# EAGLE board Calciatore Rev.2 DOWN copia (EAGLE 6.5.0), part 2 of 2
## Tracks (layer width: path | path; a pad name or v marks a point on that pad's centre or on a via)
3.3V  (via drill 0.6, 0.9 pad 1.68)  (4 unrouted)
  Top 0.305: 25.76,91.66 C23.1 | 207.73,96.14 R2.2 | C24.1 152.65,135.63 | 94.83,136.49 v94.7,136.36
  Top 0.813: C6.1 184.33,93.38 DX.BW | 207.73,96.14 207.73,97.37 v209,98.64 | v182.97,127.22 183.6,126.58 v183.6,116.42 182.53,115.35 182.53,107.91 C58.+ | v182.97,139.28 182.97,142.46 | 182.97,142.46 v182.97,144.36 | 182.97,142.46 181.7,142.46 v175.35,148.81 | v175.35,148.81 174.58,149.57 151.22,149.57 v150.84,149.95 125.69,149.95 v125.18,149.44 | 152.65,135.63 154.39,137.38 163.92,137.38 v175.35,148.81 | v125.82,142.46 124.55,141.19 v118.2,141.19 | v113.75,136.11 v106.39,136.11 106.13,135.85 106.13,133.92 | 106.13,133.92 104.5,133.92 | 104.5,133.92 102.32,136.11 99.15,136.11 | 94.83,136.49 98.77,136.49 99.15,136.11 | 104.5,133.92 104.7,133.72 C25.1 106.13,133.92 | 99.15,136.11 v99.15,130.39 | v104.23,129.12 v108.04,129.12 | v83.65,139.41 v83.65,142.2 | v80.1,142.46 74.98,142.46 AX.BW | v42.63,146.9 v40.09,149.44 38.82,149.44 v31.84,142.46 | v29.3,127.85 28.03,126.58 v28.03,124.68 | SX.BW 25.26,116.2 22.95,113.88 v22.95,106.9 22.95,106.04 25.49,103.5 | SX.VCC 25.49,103.5 | 25.49,103.5 25.26,103.5 23.58,101.82 23.58,94.66 | 23.58,94.66 C23.1 | 23.58,94.66 17.06,94.66 12.79,90.39 12.79,89.04 D11.2 | D12.2 12.86,71.9 18.5,66.26 18.5,60.54 25.49,53.56 39.46,53.56 | 39.46,53.56 44.94,53.56 v45.36,53.97 | v45.36,51.43 v45.36,53.97 | v45.36,53.97 v45.36,56.51 v45.36,59.05 | v65.49,34.51 42.63,34.51 37.55,39.59 37.55,51.65 39.46,53.56 | 154.71,67.21 148.04,73.88 142.96,73.88 139.15,77.69 139.15,86.58 138.09,87.64 PDX.VDD 112.91,87.64 TEENSY3.2_1.3.3V1 | PWR.3 158.51,71.01 154.71,67.21 | 154.71,67.21 152.87,65.37 v152.87,58.89 | PX.BW 98.7,24.53 99.78,25.62 99.78,44.67 v97.88,46.57 | v97.24,54.19 TEENSY3.2_1.3.3V
  Top 0.813: v64.22,85.94 64.22,77.64 63.87,77.28 63.87,75.6 IC2.24
  Top 1: U$10.VOUT 184.22,92.34 C6.1
  Bottom 0.305: R39.2 166.06,64.59 PWR.3 | ASX.VDD 75.1,127.13 | 196.44,107.8 R37.2 195.03,107.8 | 152.84,58.61 v152.87,58.89 | 28.03,143.73 28.03,144.04 R19.2 | 184.24,146.27 184.95,146.27 R33.2 | 83.27,144.33 R49.2 | 106.18,137.42 R23.2 106.13,138.01 | 117.56,143.38 R25.2
  Bottom 0.813: U$10.VOUT 184.22,68.78 183.6,68.16 183.6,65.38 R39.2 | DX.BW 187,98.42 182.66,102.76 182.66,102.78 182.53,102.91 182.53,107.87 C58.+ | 195.03,107.8 191.71,111.12 DX.VCC 191,111.12 193.13,113.25 193.13,116.42 | v209,98.64 209.64,99.28 209.64,110.71 203.92,116.42 193.13,116.42 | v183.6,116.42 193.13,116.42 | R35.2 183.8,128.05 | 183.8,128.05 v182.97,127.22 | 183.8,128.05 183.8,138.45 v182.97,139.28 | v182.97,144.36 183.05,144.36 R33.2 | v175.35,148.81 174.08,150.08 174.08,162.17 R31.2 | v150.84,149.95 150.84,152.29 R29.2 | v125.18,149.44 125.18,143.09 v125.82,142.46 129.63,142.46 130.26,143.09 130.26,144.97 R27.2 | R25.2 117.56,143.61 117.56,141.82 v118.2,141.19 118.2,140.55 v113.75,136.11 | v106.39,136.11 106.39,137.22 106.18,137.42 | R51.2 94.7,142.3 v94.7,136.36 86.7,136.36 v83.65,139.41 | v99.15,130.39 100.42,129.12 v104.23,129.12 | v108.04,129.12 109.31,130.39 119.47,130.39 | 119.47,130.39 124.55,130.39 135.34,119.6 136.39,119.6 ADX.VDD | QUANTUM_CONNECTOR.26 120.21,129.65 119.47,130.39 | v83.65,142.2 83.65,143.73 | 83.65,143.73 83.65,143.95 83.27,144.33 | v80.1,142.46 82,142.46 83.27,143.73 83.65,143.73 | AX.BW 74.57,142.91 72.48,145 63.99,145 AX.VCC 57.83,146.9 v42.63,146.9 | 64.23,145.23 R47.2 | R21.2 38.7,159.72 40.09,158.33 v40.09,149.44 | v31.84,142.46 29.61,142.46 | 29.61,142.46 R19.2 | 29.61,142.46 29.61,128.16 v29.3,127.85 | R17.2 22.17,124.68 v28.03,124.68 28.03,117.92 SX.BW | v22.95,106.9 20.99,106.9 R15.2 | D11.2 D13.2 D30.2 D6.2 D12.2 | v45.36,59.05 45.36,59.72 42,63.08 32.85,63.08 R13.2 | R45.2 64.45,30.92 66.13,32.6 66.13,33.87 v65.49,34.51 | 152.84,58.61 R41.2
  Bottom 0.813: v97.88,46.57 97.24,47.21 v97.24,54.19 | PX.BW 98.7,22.26 99.15,21.81 109.31,21.81 | 109.31,21.81 109.71,21.81 PX.VCC | R43.2 108.78,21.28 109.31,21.81 | 73.75,142.05 73.75,128.98 ASX.VDD | 75.1,127.13 74.93,127.13 73.11,125.31 73.11,111.34 77.56,106.9 77.56,96.1 76.92,95.47 75.69,95.47 PSX.VDD 68.58,95.38 64.22,91.02 v64.22,85.94
5V  (via drill 0.6)
  Top 0.305: QUANTUM_CONNECTOR.25 120.21,123.3 147.41,96.1 147.41,92.13 C15.+
  Top 0.813: v180.43,72.61 181.7,72.61 187.41,78.32 v195.67,78.32 | v198.21,94.2 198.21,94.83 199.48,96.1 201.47,96.1 R3.2
  Bottom 0.813: 158.39,77.24 IC1.3 158.39,81.15 C15.+ | 158.39,77.24 156.93,75.78 155.03,75.78 153.76,74.51 153.76,72.46 PWR.1 | 158.39,77.24 170.08,77.24 174.71,72.61 v180.43,72.61 | v195.67,78.32 196.3,78.32 198.21,80.23 v198.21,94.2
BATLVL  (via drill 0.6)
  Top 0.305: TP1.TP 205.99,72.77 203.92,70.7 171.54,70.7 171.54,70.57 149.69,48.73 | 149.69,48.73 98.26,48.73 95.97,51.02 v95.97,59.91 | TEENSY3.2_1.32 104.67,74.51 102.96,74.51 101.56,73.11 96.35,73.11 94.7,71.46 94.7,65.24 v95.34,64.61 | R6.2 133.32,73.48 R5.1 136.97,72.89 138.52,71.34 146.14,71.34 149.31,68.16 149.69,67.78 149.69,48.73
  Bottom 0.305: v95.34,64.61 95.34,63.72 95.97,63.08 v95.97,59.91
BLUE(RGB)  (via drill 0.6)
  Top 0.305: v128.99,129.76 127.09,129.76 125.18,127.85 115.02,127.85 113.88,126.71 113.88,122.26 108.67,117.06 90.26,117.06 v89.62,116.42 | v143.6,141.19 147.77,141.19 R-B.1
  Bottom 0.305: v128.99,129.76 140.42,141.19 v143.6,141.19 | v89.62,116.42 89.62,115.15 106.13,98.64 107.4,98.64 120.1,85.94 120.1,67.53 119.47,66.89 115.02,66.89 TEENSY3.2_1.5
BUZZER
  Bottom 0.305: TEENSY3.2_1.RESET/DAC 102.32,84.67 102.32,91.02 87.08,106.26 86.45,106.26 80.1,99.91 80.1,94.83 79.46,94.2 79.46,82.13 76.29,78.96 75.02,78.96 74.38,79.59 74.38,87.21 72.07,89.53 BUZZER.+
CS1
  Top 0.305: IC2.22 66.31,77.24 68.67,79.59 68.67,85.94 72.48,89.75 72.48,118.33 73.75,119.6 75.51,119.6 ASX.CS
CS2  (via drill 0.6)
  Top 0.305: IC2.21 67.58,76.6 69.3,78.32 69.3,85.31 73.11,89.12 73.11,106.26 v73.75,106.9 | v71.21,106.9 71.84,107.53 71.84,118.96 74.38,121.5 74.38,127.85 74.94,128.41 78.12,128.41 80.73,131.03 80.73,135.47 82.64,137.38 107.4,137.38 108.04,138.01 135.34,138.01 139.79,133.57 139.79,130.14 ADX.CS
  Bottom 0.305: v73.75,106.9 v71.21,106.9
CS3  (via drill 0.6)
  Top 0.305: IC2.20 68.85,76.6 69.94,77.69 69.94,84.67 73.75,88.48 73.75,90.39 75.02,91.66 76.29,91.66 78.83,94.2 78.83,99.91 85.18,106.26 85.18,108.8 v91.53,115.15 | PDX.CS 135.8,96.1 v134.07,96.1
  Bottom 0.305: v134.07,96.1 133.44,96.74 110.58,96.74 108.04,99.28 106.77,99.28 91.53,114.52 v91.53,115.15
CS4
  Top 0.305: IC2.19 70.12,76.6 70.57,77.05 70.57,84.04 74.38,87.85 75.52,87.85 PSX.CS
D+
  Bottom 0.305: USB_2.3 84.54,32.6 87.72,35.78 104.23,35.78 106.13,37.68 USB.2
D-
  Bottom 0.305: USB.1 103.59,37.68 102.32,36.41 87.08,36.41 82,31.33 USB_2.2
EXP-READ-1  (via drill 0.6)
  Top 0.305: TEENSY3.2_1.14/A0 99.59,82.13 v83.91,82.13 | v80.1,75.15 v80.1,68.16 | v69.3,68.16 68.03,69.43 66.76,69.43 64.86,67.53 64.22,67.53 63.77,67.08 IC2.1
  Bottom 0.305: v83.91,82.13 82.64,80.86 82.64,78.96 80.1,76.42 v80.1,75.15 | v80.1,68.16 79.46,67.53 69.3,67.53 v69.3,68.16
EXPA
  Top 0.305: IC2.10 75.2,63.72 75.96,62.95 96.1,62.95 98.51,60.54 100.42,60.54 101.05,59.91 101.05,58.64 102.96,56.73 111.21,56.73 111.85,57.37 111.85,58.64 112.48,59.27 114.83,59.27 TEENSY3.2_1.2
EXPB
  Top 0.305: IC2.11 76.47,64.35 77.23,63.59 97.37,63.59 98,62.95 113.69,62.95 TEENSY3.2_1.3
EXPC  (via drill 0.6)
  Top 0.305: IC2.14 76.47,74.33 v77.56,73.24 | v102.96,75.78 108.67,75.78 109.05,75.78 109.31,75.78 111.21,73.88 111.21,70.07 112.48,68.8 112.48,66.26 114.48,64.25 TEENSY3.2_1.4
  Bottom 0.305: v77.56,73.24 100.42,73.24 v102.96,75.78
EXPD  (via drill 0.6)
  Top 0.305: TEENSY3.2_1.24 107.4,71.97 108.67,71.97 109.94,70.7 109.94,64.99 109.31,64.35 105.5,64.35 102.96,66.89 v102.32,66.89 | IC2.13 78.65,76.42 80.73,76.42 82,75.15 v82,68.16 | v101.69,69.43 101.69,70.07 101.05,70.7 v95.97,70.7
  Bottom 0.305: v102.32,66.89 101.69,67.53 v101.69,69.43 | v82,68.16 82.64,67.53 93.43,67.53 95.97,70.07 v95.97,70.7
GND  (via drill 0.6, 1.1)
  Top 0.305: v112.48,40.22 112.48,39.59 111.21,38.32 USB.3 | C25.2 108.73,132.99 108.17,132.99 106.89,131.71 102.91,131.71 101.05,133.57 v101.05,134.76
  Top 0.406: v72.48,80.86 75.19,78.14 IC2.15
  Bottom 0.305: C51.2 63.22,28.49 62.72,28.99 62.72,31.53 C52.1 | TEENSY3.2_1.GND 108.57,51.55 108.04,50.38 108.04,44.67 v112.48,40.22 | v101.05,134.76 101.05,136.74 99.78,138.01 98.51,138.01 97.24,139.28 97.24,142.51 C22.1 | C29.1 117.87,146.06 C28.2
  Bottom 0.406: BUZZER.- 59.33,88.3 65.49,82.13 71.21,82.13 v72.48,80.86
  other vias: 45.43,48.98 45.43,46.57 45.43,43.9 45.43,41.24
  pour Top (isolate 0.406): -25.31,195.8 245.83,192.62 245.83,-21.37 -25.31,-18.2
  pour Bottom (isolate 0.406): -19.6,197.07 258.53,195.8 258.53,-19.47 -19.6,-18.2
GREEN(RGB)  (via drill 0.6)
  Top 0.305: v127.09,132.93 114.64,132.93 108.8,127.09 108.8,122.26 104.86,118.33 v85.18,118.33 | v138.52,146.9 147.91,146.9 R-G.1
  Bottom 0.305: v127.09,132.93 137.25,143.09 137.25,145.63 v138.52,146.9 | v85.18,118.33 85.18,117.06 104.86,97.37 106.13,97.37 118.83,84.67 118.83,71.97 116.19,69.33 TEENSY3.2_1.6
INA1-31-2
  Top 0.305: ASX.INA 75.59,111.92 77.56,113.88 77.56,123.41 82,127.85 87.93,127.85 QUANTUM_CONNECTOR.2
INA2-32-2
  Top 0.305: ADX.INA 112.88,134.6 109.31,131.03 102.32,131.03 QUANTUM_CONNECTOR.8
INA3-33-2
  Bottom 0.305: 136.43,103.09 PDX.INA 135.77,102.88 135.34,102.45 135.34,99.28 134.71,98.64 112.48,98.64 109.94,101.18 108.67,101.18 94.7,115.15 94.7,115.79 QUANTUM_CONNECTOR.11
INA4-34-2  (via drill 0.6)
  Top 0.305: QUANTUM_CONNECTOR.5 | QUANTUM_CONNECTOR.5 90.89,119.6 80.73,119.6 80.1,118.96 80.1,113.25 83.91,109.44 v83.91,108.8
  Bottom 0.305: 84.54,108.8 v83.91,108.8 85.18,107.53 85.18,106.26 79.46,100.55 79.46,95.47 78.83,94.83 78.83,83.4 75.61,80.18 PSX.INA
INB1-35-2
  Top 0.305: QUANTUM_CONNECTOR.6 94.81,127.74 93.43,129.12 80.12,129.12 ASX.INB
INB2-36-2
  Bottom 0.305: ADX.INB 134.31,121.9 122.64,133.57 115.66,133.57 113.75,131.66 108.67,131.66 104.86,127.85 104.23,127.85 QUANTUM_CONNECTOR.12
INB3-37-2
  Bottom 0.305: 136.43,90.39 PDX.INB 135.34,91.48 135.34,96.74 134.71,97.37 111.21,97.37 108.67,99.91 107.4,99.91 92.8,114.52 92.8,118.96 QUANTUM_CONNECTOR.7
INB4-38-2
  Top 0.305: PSX.INB 75.61,92.88 78.19,95.47 78.19,121.5 81.37,124.68 88.57,124.68 QUANTUM_CONNECTOR.1
LED1  (via drill 0.6)
  Top 0.305: LED4.A 119.62,3.87 118.83,4.66 v118.83,7.84 | 115.02,77.05 TEENSY3.2_1.9 116.1,75.78 v121.37,75.78 | v125.18,58 125.18,75.15 v124.55,75.78
  Bottom 0.305: v118.83,7.84 118.83,51.65 v125.18,58 | v124.55,75.78 v121.37,75.78
LED2  (via drill 0.6)
  Top 0.305: LED2.A 124.39,3.87 122.64,2.12 120.1,2.12 117.56,4.66 v117.56,5.93 | TEENSY3.2_1.10 116.73,77.69 122.64,77.69 123.28,77.05 v123.28,58
  Bottom 0.305: v117.56,5.93 117.56,8.47 118.2,9.11 118.2,52.92 v123.28,58
LED_ALIM  (via drill 0.6)
  Top 0.305: TEENSY3.2_1.31 106.13,78.32 109.94,78.32 111.85,76.42 111.85,70.7 114.39,68.16 v122.01,68.16 | R8.1 127.25,68.96 v127.09,68.8
  Bottom 0.305: v127.09,68.8 122.64,68.8 v122.01,68.16
MISO_12  (via drill 0.6)
  Top 0.305: v27.39,73.88 43.9,73.88 48.98,78.96 60.41,78.96 v61.05,79.59 | v86.45,104.36 100.42,104.36 110.58,94.2 v110.58,91.02
  Bottom 0.305: D12.3 15.52,73.88 v27.39,73.88 | v61.05,79.59 64.86,79.59 65.49,78.96 73.75,78.96 74.38,78.32 76.92,78.32 80.1,81.5 80.1,93.56 80.73,94.2 80.73,99.28 85.81,104.36 v86.45,104.36 | v110.58,91.02 111.21,91.02 115.02,87.21 115.02,84.67 TEENSY3.2_1.12
MOSI_11  (via drill 0.6)
  Top 0.305: v40.73,70.7 42,70.7 49.62,78.32 v62.32,78.32 | v85.81,102.45 85.18,103.09 85.18,104.99 85.81,105.63 87.08,105.63 87.72,104.99 101.05,104.99 111.85,94.2 111.85,90.39 v110.58,89.12
  Bottom 0.305: D11.3 18,88.98 36.28,70.7 v40.73,70.7 | v62.32,78.32 73.11,78.32 73.75,77.69 77.56,77.69 80.73,80.86 80.73,92.93 81.37,93.56 81.37,98.01 v85.81,102.45 | v110.58,89.12 111.85,89.12 113.75,87.21 113.75,83.21 TEENSY3.2_1.11
MOTORE1-1
  Bottom 2.184: X1.1 41.34,113.13 ASX.INMOT2
MOTORE1-2
  Bottom 2.184: X1.2 41.42,118.13 ASX.INMOT1
MOTORE2-1
  Bottom 2.184: PDX.INMOT2 166.77,101.61 X2.1
MOTORE2-2
  Bottom 2.184: PDX.INMOT1 166.75,96.53 X2.2
MOTORE3-1
  Bottom 2.184: ADX.INMOT2 166.48,133.33 X3.1
MOTORE3-2
  Bottom 2.184: ADX.INMOT1 166.5,128.25 X3.2
MOTORE4-1
  Bottom 2.184: X4.1 41.41,81.51 PSX.INMOT2
MOTORE4-2
  Bottom 2.184: X4.2 41.33,86.51 PSX.INMOT1
N$1
  Top 0.305: R1.2 LED2.C
N$2  (via drill 0.6)
  Top 0.305: R8.2 139.95,68.8 146.77,68.8 v148.04,67.53 | v167.12,63.51 173.44,69.84 204.33,69.84 207.73,73.24 207.73,84.93 LED1.A
  Bottom 0.305: v148.04,67.53 151.85,63.72 166.91,63.72 v167.12,63.51
N$3
  Bottom 0.305: 0°.VCC 103.51,148.41 C26.1 R23.1
N$4
  Bottom 0.305: R24.1 110.01,142.96 0°.OUT
N$6
  Bottom 0.305: 12°.VCC 114.91,151.03 C28.1 114.82,146.52 R25.1
N$7
  Bottom 0.305: 12°.OUT 123,146.77 R26.1
N$9
  Bottom 0.305: R13.1 C1.1 28.66,57.37 26.7,57.37 240°.VCC
N$13
  Bottom 0.305: 270°.VCC 14.19,103.37 C4.1 R15.1
N$14
  Bottom 0.305: 282°.VCC 16.95,123.48 C9.1 R17.1
N$15
  Bottom 0.305: 25°.OUT 135.4,149.25 R28.1
N$16
  Bottom 0.305: R30.1 154.39,158.97 38°.OUT
N$17
  Top 1: C5.+ 180.54,87.48 179.16,88.86 179.16,90.14 U$10.VIN U$10.SHDN 176.01,89.58 D2.C
N$18
  Bottom 0.305: 51°.OUT 182.97,162.14 R32.1
N$20
  Bottom 0.305: 25°.VCC 127.17,154.39 C30.1 127.23,148.36 R27.1
N$24
  Bottom 0.305: 295°.VCC 20.81,146.09 C11.1 R19.1
N$25
  Bottom 0.305: 308°.VCC 31.3,163.54 C13.1 R21.1
N$26
  Bottom 0.305: 321°.VCC 61.53,160.31 C17.1 61.43,155.01 R47.1
N$27
  Bottom 0.305: R34.1 191.86,143.73 194.4,145 64°.OUT
N$28
  Bottom 0.305: R29.1 C32.1 148.08,162.52 38°.VCC
N$34
  Bottom 0.305: R36.1 198.84,124.04 77°.OUT
N$35
  Bottom 0.305: 51°.VCC 177.89,168.49 C34.1 R31.1
N$36
  Bottom 0.305: R40.1 185.51,57.37 120°.OUT
N$37
  Bottom 0.305: 64°.VCC 188.68,151.35 C36.1 R33.1
N$38
  Bottom 0.305: 180°.OUT 103.17,14.14 R44.1
N$39
  Bottom 0.305: 77°.VCC 196.94,131.66 C38.1 R35.1
N$40
  Bottom 0.305: R38.1 200.53,102.69 90°.OUT
N$41
  Bottom 0.305: 90°.VCC 202.25,110.44 C43.1 195.84,110.44 R37.1
N$42
  Bottom 0.305: 150°.OUT 150.58,24.35 R42.1
N$43
  Bottom 0.305: 120°.VCC 189.95,64.35 C45.1 R39.1
N$44
  Bottom 0.305: R46.1 57.24,28.79 210°.OUT
N$45
  Bottom 0.305: 150°.VCC 157.57,26.03 157.57,28.79 C47.1 R41.1
N$51
  Bottom 0.305: R14.1 24.85,64.35 240°.OUT
N$52
  Bottom 0.305: 180°.VCC 111.62,13.78 C49.1 111.58,16.47 R43.1
N$53
  Bottom 0.305: 270°.OUT 14.13,111.44 R16.1
N$54
  Bottom 0.305: 210°.VCC 64.86,24.98 C51.1 R45.1
N$56
  Bottom 0.305: 282°.OUT R18.1
N$57
  Bottom 0.305: 295°.OUT R20.1
N$60
  Bottom 0.305: 308°.OUT 38.19,168.49 R22.1
N$64
  Top 0.305: 3.3V.A 207.74,93.19 R2.1
N$65
  Bottom 0.305: 321°.OUT 69.62,159.46 R48.1
N$67
  Top 0.305: LED_RGB.3 152.1,142.2 R-B.2
N$68
  Top 0.305: LED_RGB.1 152.26,145.6 R-G.2
N$69
  Top 0.305: R7.2 LED4.C
N$81
  Top 0.305: LED_RGB.2 150.91,143.9 R-R.2
N$95
  Top 0.305: C14.+ 149.75,82.92 IC1.1 153.25,79.31 153.25,78.19
  Top 0.813: 153.25,78.19 155.66,75.78 164.85,75.78 D1.C
N$97
  Top 0.305: 5V.A 201.59,93.19 R3.1
N$135  (via drill 0.9 pad 1.68)
  other vias: 75.84,41.27
N$136  (via drill 0.9 pad 1.68)
  other vias: 75.84,43.81
N$137  (via drill 0.9 pad 1.68)
  other vias: 75.84,46.35
N$138  (via drill 0.9 pad 1.68)
  other vias: 75.84,48.89
N$139  (via drill 0.9 pad 1.68)
  other vias: 75.84,51.43
N$140  (via drill 0.9 pad 1.68)
  other vias: 75.84,53.97
N$141  (via drill 0.9 pad 1.68)
  other vias: 75.84,56.51
N$142  (via drill 0.9 pad 1.68)
  other vias: 75.84,59.05
N$143  (via drill 0.9 pad 1.68)
  other vias: 98.51,14.85
N$144  (via drill 0.9 pad 1.68)
  other vias: 98.51,17.39
N$145  (via drill 0.9 pad 1.68)
  other vias: 98.51,19.93
N$146  (via drill 0.9 pad 1.68)
  other vias: 95.97,19.93
N$147  (via drill 0.9 pad 1.68)
  other vias: 95.97,17.39
N$148  (via drill 0.9 pad 1.68)
  other vias: 95.97,14.85
N$149  (via drill 0.9 pad 1.68)
  other vias: 70.76,59.05
N$150  (via drill 0.9 pad 1.68)
  other vias: 73.3,59.05
N$151  (via drill 0.9 pad 1.68)
  other vias: 73.3,56.51
N$152  (via drill 0.9 pad 1.68)
  other vias: 70.76,56.51
N$153  (via drill 0.9 pad 1.68)
  other vias: 70.76,53.97
N$154  (via drill 0.9 pad 1.68)
  other vias: 73.3,53.97
N$155  (via drill 0.9 pad 1.68)
  other vias: 73.3,51.43
N$156  (via drill 0.9 pad 1.68)
  other vias: 70.76,51.43
N$157  (via drill 0.9 pad 1.68)
  other vias: 70.76,48.89
N$158  (via drill 0.9 pad 1.68)
  other vias: 73.3,48.89
N$159  (via drill 0.9 pad 1.68)
  other vias: 73.3,46.35
N$160  (via drill 0.9 pad 1.68)
  other vias: 70.76,46.35
N$161  (via drill 0.9 pad 1.68)
  other vias: 70.76,43.81
N$162  (via drill 0.9 pad 1.68)
  other vias: 73.3,43.81
N$163  (via drill 0.9 pad 1.68)
  other vias: 73.3,41.27
N$165  (via drill 0.9 pad 1.68)
  other vias: 70.76,41.27
N$171  (via drill 0.9 pad 1.68)
  other vias: 68.22,41.27
N$172  (via drill 0.9 pad 1.68)
  other vias: 68.22,43.81
N$173  (via drill 0.9 pad 1.68)
  other vias: 68.22,46.35
N$174  (via drill 0.9 pad 1.68)
  other vias: 68.22,48.89
N$175  (via drill 0.9 pad 1.68)
  other vias: 68.22,51.43
N$176  (via drill 0.9 pad 1.68)
  other vias: 68.22,53.97
N$177  (via drill 0.9 pad 1.68)
  other vias: 68.22,56.51
N$178  (via drill 0.9 pad 1.68)
  other vias: 68.22,59.05
N$179  (via drill 0.9 pad 1.68)
  other vias: 93.43,14.85
N$180  (via drill 0.9 pad 1.68)
  other vias: 93.43,17.39
N$181  (via drill 0.9 pad 1.68)
  other vias: 93.43,19.93
N$182  (via drill 0.9 pad 1.68)
  other vias: 90.89,19.93
N$183  (via drill 0.9 pad 1.68)
  other vias: 90.89,17.39
N$184  (via drill 0.9 pad 1.68)
  other vias: 90.89,14.85
N$185  (via drill 0.9 pad 1.68)
  other vias: 65.68,59.05
N$186  (via drill 0.9 pad 1.68)
  other vias: 65.68,56.51
N$187  (via drill 0.9 pad 1.68)
  other vias: 65.68,53.97
N$188  (via drill 0.9 pad 1.68)
  other vias: 65.68,51.43
N$189  (via drill 0.9 pad 1.68)
  other vias: 65.68,48.89
N$190
  Bottom 0.305: 334°.VCC 80.79,150.52 C19.1 80.89,147.95 R49.1
N$191
  Bottom 0.305: 347°.VCC 92.32,147.24 C21.1 92.32,142.72 R51.1
N$192  (via drill 0.9 pad 1.68)
  other vias: 65.68,46.35
N$193  (via drill 0.9 pad 1.68)
  other vias: 65.68,43.81
N$194  (via drill 0.9 pad 1.68)
  other vias: 65.68,41.27
N$197  (via drill 0.9 pad 1.68)
  other vias: 88.35,14.85
N$198  (via drill 0.9 pad 1.68)
  other vias: 88.35,17.39
N$199  (via drill 0.9 pad 1.68)
  other vias: 88.35,19.93
N$201
  Bottom 0.305: 334°.OUT 88.77,153.6 R50.1
N$202
  Bottom 0.305: R52.1 100.25,151.21 arc90 347°.OUT
N$203  (via drill 0.9 pad 1.68)
  other vias: 85.81,19.93
N$204  (via drill 0.9 pad 1.68)
  other vias: 85.81,17.39
N$205  (via drill 0.9 pad 1.68)
  other vias: 85.81,14.85
N$207  (via drill 0.9 pad 1.68)
  other vias: 60.6,59.05
N$208  (via drill 0.9 pad 1.68)
  other vias: 63.14,59.05
N$209  (via drill 0.9 pad 1.68)
  other vias: 63.14,56.51
N$210  (via drill 0.9 pad 1.68)
  other vias: 60.6,56.51
N$211  (via drill 0.9 pad 1.68)
  other vias: 60.6,53.97
N$214  (via drill 0.9 pad 1.68)
  other vias: 63.14,53.97
N$215  (via drill 0.6)
  Top 0.305: v196.3,58.64 166.23,28.57 109.66,28.57 R4.1 | v202.65,101.82 196.14,101.82 DX.TX
  Bottom 0.305: v196.3,58.64 196.3,66.89 201.38,71.97 204.56,71.97 205.19,72.61 205.19,99.28 v202.65,101.82
N$216  (via drill 0.9 pad 1.68)
  other vias: 63.14,51.43
N$217  (via drill 0.9 pad 1.68)
  other vias: 60.6,51.43
N$218  (via drill 0.9 pad 1.68)
  other vias: 60.6,48.89
N$219  (via drill 0.9 pad 1.68)
  other vias: 63.14,48.89
N$220  (via drill 0.9 pad 1.68)
  other vias: 63.14,46.35
N$221  (via drill 0.9 pad 1.68)
  other vias: 60.6,46.35
N$222  (via drill 0.9 pad 1.68)
  other vias: 60.6,43.81
N$223  (via drill 0.9 pad 1.68)
  other vias: 63.14,43.81
N$224  (via drill 0.9 pad 1.68)
  other vias: 63.14,41.27
N$226  (via drill 0.9 pad 1.68)
  other vias: 60.6,41.27
N$235  (via drill 0.9 pad 1.68)
  other vias: 58.06,41.27
N$236  (via drill 0.9 pad 1.68)
  other vias: 58.06,43.81
N$237  (via drill 0.9 pad 1.68)
  other vias: 58.06,46.35
N$238  (via drill 0.9 pad 1.68)
  other vias: 58.06,48.89
N$241  (via drill 0.9 pad 1.68)
  other vias: 58.06,51.43
N$242  (via drill 0.9 pad 1.68)
  other vias: 58.06,53.97
N$243  (via drill 0.9 pad 1.68)
  other vias: 58.06,56.51
N$244  (via drill 0.9 pad 1.68)
  other vias: 58.06,59.05
N$245  (via drill 0.9 pad 1.68)
  other vias: 83.27,14.85
N$246  (via drill 0.9 pad 1.68)
  other vias: 83.27,17.39
N$247  (via drill 0.9 pad 1.68)
  other vias: 83.27,19.93
N$248  (via drill 0.9 pad 1.68)
  other vias: 80.73,19.93
N$249  (via drill 0.9 pad 1.68)
  other vias: 80.73,17.39
N$250  (via drill 0.9 pad 1.68)
  other vias: 80.73,14.85
N$251  (via drill 0.9 pad 1.68)
  other vias: 55.52,59.05
N$252  (via drill 0.9 pad 1.68)
  other vias: 55.52,56.51
N$253  (via drill 0.9 pad 1.68)
  other vias: 55.52,53.97
N$254  (via drill 0.9 pad 1.68)
  other vias: 55.52,51.43
N$255  (via drill 0.9 pad 1.68)
  other vias: 55.52,48.89
N$256  (via drill 0.9 pad 1.68)
  other vias: 55.52,46.35
N$257  (via drill 0.9 pad 1.68)
  other vias: 55.52,43.81
N$258  (via drill 0.9 pad 1.68)
  other vias: 55.52,41.27
N$263  (via drill 0.9 pad 1.68)
  other vias: 52.98,41.27
N$264  (via drill 0.9 pad 1.68)
  other vias: 52.98,43.81
N$265  (via drill 0.9 pad 1.68)
  other vias: 52.98,46.35
N$266  (via drill 0.9 pad 1.68)
  other vias: 52.98,48.89
N$267  (via drill 0.9 pad 1.68)
  other vias: 52.98,51.43
N$268  (via drill 0.9 pad 1.68)
  other vias: 52.98,53.97
N$269  (via drill 0.9 pad 1.68)
  other vias: 52.98,56.51
N$270  (via drill 0.9 pad 1.68)
  other vias: 52.98,59.05
N$271  (via drill 0.9 pad 1.68)
  other vias: 78.19,14.85
N$272  (via drill 0.9 pad 1.68)
  other vias: 78.19,17.39
N$273  (via drill 0.9 pad 1.68)
  other vias: 78.19,19.93
N$315  (via drill 0.9 pad 1.68)
  other vias: 75.65,19.93
N$316  (via drill 0.9 pad 1.68)
  other vias: 75.65,17.39
N$317  (via drill 0.9 pad 1.68)
  other vias: 75.65,14.85
N$318  (via drill 0.9 pad 1.68)
  other vias: 50.44,59.05
N$319  (via drill 0.9 pad 1.68)
  other vias: 50.44,56.51
N$320  (via drill 0.9 pad 1.68)
  other vias: 50.44,53.97
N$321  (via drill 0.9 pad 1.68)
  other vias: 50.44,51.43
N$322  (via drill 0.9 pad 1.68)
  other vias: 50.44,48.89
N$323  (via drill 0.9 pad 1.68)
  other vias: 50.44,46.35
N$324  (via drill 0.9 pad 1.68)
  other vias: 50.44,43.81
N$325  (via drill 0.9 pad 1.68)
  other vias: 50.44,41.27
N$330  (via drill 0.9 pad 1.68)
  other vias: 47.9,41.27
N$331  (via drill 0.9 pad 1.68)
  other vias: 47.9,43.81
N$332  (via drill 0.9 pad 1.68)
  other vias: 47.9,46.35
N$333  (via drill 0.9 pad 1.68)
  other vias: 47.9,48.89
N$334  (via drill 0.9 pad 1.68)
  other vias: 47.9,51.43
N$335  (via drill 0.9 pad 1.68)
  other vias: 47.9,53.97
N$336  (via drill 0.9 pad 1.68)
  other vias: 47.9,56.51
N$337  (via drill 0.9 pad 1.68)
  other vias: 47.9,59.05
N$338  (via drill 0.9 pad 1.68)
  other vias: 73.11,14.85
N$339  (via drill 0.9 pad 1.68)
  other vias: 73.11,17.39
N$340  (via drill 0.9 pad 1.68)
  other vias: 73.11,19.93
N$341  (via drill 0.9 pad 1.68)
  other vias: 70.57,19.93
N$342  (via drill 0.9 pad 1.68)
  other vias: 70.57,17.39
N$343  (via drill 0.9 pad 1.68)
  other vias: 70.57,14.85
NC
  Top 0.305: TEENSY3.2_1.8 TEENSY3.2_1.7
PROGRAM  (via drill 0.6)
  Top 0.305: v107.4,35.78 109.94,35.78 114.39,40.22 114.39,41.49 113.75,42.13 106.59,42.13 v105.95,42.76
  Bottom 0.305: TEENSY3.2_1.PGM 104.77,84.08 105.95,82.89 v105.95,42.76 | USB_2.5 89.62,34.51 90.26,35.14 106.77,35.14 v107.4,35.78
PWM1-2
  Top 0.305: QUANTUM_CONNECTOR.4 92.27,127.74 91.53,128.49 81.37,128.49 76.92,124.04 76.92,118.3 ASX.PWM
PWM2-2
  Top 0.305: ADX.PWM 136.47,129.52 132.04,133.95 113.5,133.95 109.94,130.39 102.96,130.39 99.78,127.22 99.78,126.16 QUANTUM_CONNECTOR.10
PWM3-2
  Bottom 0.305: PDX.PWM 136.43,98.01 111.85,98.01 109.31,100.55 108.04,100.55 93.43,115.15 93.43,117.06 QUANTUM_CONNECTOR.9
PWM4-2  (via drill 0.6)
  Top 0.305: QUANTUM_CONNECTOR.3 92.27,122.24 90.26,120.23 80.1,120.23 79.46,119.6 79.46,112.61 82.64,109.44 82.64,108.17 v83.91,106.9
  Bottom 0.305: PSX.PWM 76.2,85.22 78.19,87.21 78.19,95.47 78.83,96.1 78.83,101.82 v83.91,106.9
RED(RGB)  (via drill 0.6)
  Top 0.305: R-R.1 v140.03,143.97 | v128.74,131.66 125.82,131.66 125.18,132.3 116.29,132.3 111.34,127.34 111.34,122.26 106.77,117.69 87.72,117.69 v87.08,117.06 | v111.21,68.16 110.58,68.8 110.58,73.24 109.31,74.51 107.4,74.51 TEENSY3.2_1.25
  Bottom 0.305: v128.74,131.66 128.99,131.66 138.52,141.19 138.52,142.46 v140.03,143.97 | v87.08,117.06 87.08,116.42 105.5,98.01 106.77,98.01 119.47,85.31 119.47,70.07 117.56,68.16 v111.21,68.16
S1-A0  (via drill 0.6)
  Top 0.305: TEENSY3.2_1.15/A1 101.05,80.86 101.05,82.77 100.42,83.4 98.51,83.4 98.51,85.94 102.32,89.75 107.4,89.75 108.04,90.39 v108.04,93.56
  Bottom 0.305: R24.2 C27.1 111.58,135.84 109.31,133.57 80.1,133.57 79.46,132.93 79.46,118.96 104.86,93.56 v108.04,93.56
S2-A1  (via drill 0.6)
  Top 0.305: v106.77,94.83 106.77,91.02 106.13,90.39 101.69,90.39 v95.97,84.67
  Bottom 0.305: R26.2 C29.2 122.97,143.42 112.48,132.93 80.73,132.93 80.1,132.3 80.1,119.6 104.86,94.83 v106.77,94.83 | v95.97,84.67 95.97,78.32 97.34,76.95 TEENSY3.2_1.16/A2
S3-A2  (via drill 0.6)
  Top 0.305: v105.5,96.1 105.5,91.66 104.86,91.02 100.42,91.02 v99.78,90.39
  Bottom 0.305: R28.2 C31.2 135.59,143.97 132.8,141.19 122.01,141.19 113.12,132.3 81.37,132.3 80.73,131.66 80.73,120.23 104.86,96.1 v105.5,96.1 | TEENSY3.2_1.17/A3 101.05,75.78 101.05,89.75 100.42,90.39 v99.78,90.39
S4-A3  (via drill 0.6)
  Top 0.305: TEENSY3.2_1.18/A4 102.35,71.87 103.59,73.11 v108.8,73.11 | v117.56,73.24 v122.01,73.24
  Bottom 0.305: R30.2 C33.2 155.96,128.49 137.88,110.41 137.88,76.29 134.83,73.24 v122.01,73.24 | v108.8,73.11 109.18,73.24 v117.56,73.24
S5-A4  (via drill 0.6)
  Top 0.305: v104.86,61.81 v108.67,61.81
  Bottom 0.305: R32.2 C35.2 178.02,149.44 138.52,109.94 138.52,68.16 134.71,64.35 125.18,64.35 124.55,64.99 117.56,64.99 115.66,63.08 110.58,63.08 109.31,61.81 v108.67,61.81 | TEENSY3.2_1.19/A5 99.69,68.89 100.32,68.89 101.05,68.16 101.05,66.26 101.69,65.62 102.96,65.62 103.59,64.99 103.59,63.72 104.86,62.45 v104.86,61.81
S6-A5  (via drill 0.6)
  Top 0.305: v133.94,65.49 v137.88,65.49 | TEENSY3.2_1.20/A6 100.86,65.62 102.96,65.62 104.86,63.72 110.58,63.72 111.08,64.22 v111.08,65.49
  Bottom 0.305: R34.2 C37.2 171.12,141.4 139.15,109.44 139.15,66.76 v137.88,65.49 | v133.94,65.49 v111.08,65.49
S7-A6  (via drill 0.6)
  Top 0.305: v104.35,59.27 v108.67,59.27
  Bottom 0.305: R36.2 C42.2 174.95,122.63 172.93,120.61 151.6,120.61 139.79,108.8 139.79,65.62 136.61,62.45 118.07,62.45 116.16,60.54 113.75,60.54 112.48,59.27 v108.67,59.27 | TEENSY3.2_1.21/A7 100.86,63.08 102.96,63.08 103.46,62.57 103.46,60.16 v104.35,59.27
S8-A7  (via drill 0.6)
  Top 0.305: v97.37,56.55 v97.37,58.76 | v103.46,57.87 v110.58,57.87
  Bottom 0.305: v103.46,57.87 100.92,55.33 97.98,55.33 97.37,55.94 v97.37,56.55 | v97.37,58.76 97.37,59.4 TEENSY3.2_1.22/A8 | v110.58,57.87 115.66,57.87 119.59,61.81 137.25,61.81 140.42,64.99 140.42,93.56 141.06,94.2 146.77,94.2 147.41,94.83 147.41,97.37 148.68,98.64 162.01,98.64 163.54,97.12 163.54,93.94 173.06,93.94 174.58,95.47 190.59,95.47 195.7,100.58 C44.2 198.38,104.85 R38.2
S9-A8  (via drill 0.6)
  Top 0.305: IC2.9 73.93,63.08 74.69,62.32 95.72,62.32 98.77,59.27 99.59,59.27 TEENSY3.2_1.23/A9 99.69,58.73 105.5,52.92 v108.67,52.92
  Bottom 0.305: R40.2 C46.2 123.32,59.95 116.29,52.92 v108.67,52.92
S10-A9  (via drill 0.6)
  Top 0.305: IC2.8 72.66,62.45 73.42,61.68 92.42,61.68 94.07,60.03 94.07,47.84 97.88,44.03 v97.88,33.24 | v144.87,30.06 144.23,29.43 111.85,29.43 110.58,30.7 104.23,30.7 v101.69,33.24
  Bottom 0.305: R42.2 C48.2 148.13,30.06 v144.87,30.06 | v97.88,33.24 v101.69,33.24
S11-A10  (via drill 0.6)
  Top 0.305: IC2.7 71.39,61.81 72.15,61.05 91.91,61.05 93.43,59.53 93.43,47.21 96.61,44.03 v96.61,25.62
  Bottom 0.305: R44.2 103.32,18.95 C50.2 100.43,19.28 99.78,18.63 97.88,18.63 97.24,19.27 97.24,24.98 v96.61,25.62
S12-A11  (via drill 0.6)
  Top 0.305: IC2.6 70.12,61.18 70.88,60.41 91.4,60.41 92.8,59.02 92.8,46.57 95.34,44.03 v95.34,37.68
  Bottom 0.305: R46.2 C52.2 64,37.05 94.7,37.05 v95.34,37.68
S13-A12  (via drill 0.6)
  Top 0.305: IC2.5 68.85,63.27 v68.67,63.08
  Bottom 0.305: R14.2 C2.2 32.79,69.11 35.65,66.26 43.9,66.26 45.81,64.35 67.4,64.35 v68.67,63.08
S14-A13
  Bottom 0.305: R16.2 C8.2 24.25,111.5 25.13,112.38 30.16,112.38 33.74,108.8 33.74,75.78 36.28,73.24 40.73,73.24 48.98,64.99 88.99,64.99 96.3,57.82 100.26,57.82 100.92,58.48 100.92,60.41 TEENSY3.2_1.A10
S15-A14
  Bottom 0.305: R18.2 C10.2 27.86,125.95 29.93,125.95 34.38,121.5 34.38,76.42 36.92,73.88 41.36,73.88 49.62,65.62 100.86,65.62 TEENSY3.2_1.A11
S16-A15  (via drill 0.6)
  Top 0.305: TEENSY3.2_1.A12 105.94,68.16 v97.5,68.16
  Bottom 0.305: R20.2 C12.2 30.37,147.73 35.01,143.09 35.01,77.05 37.55,74.51 42,74.51 50.25,66.26 95.59,66.26 v97.5,68.16
S17-A16
  Bottom 0.305: R22.2 C16.2 42.63,164.37 42.63,162.78 41.9,162.04 41.9,149.34 35.65,143.09 35.65,77.69 38.19,75.15 42.63,75.15 50.89,66.89 94.07,66.89 97.88,70.7 102.32,70.7 103.59,69.43 103.59,67.53 104.32,66.79 TEENSY3.2_1.A13
S18-A17
  Bottom 0.305: R48.2 69.72,152.16 C18.2 69.72,151.57 77.56,143.73 77.56,117.06 108.67,85.94 108.67,77.69 108.04,77.05 107.4,77.05 TEENSY3.2_1.26
S19-A18  (via drill 0.6)
  Top 0.305: v109.94,79.59 107.4,79.59 TEENSY3.2_1.27
  Bottom 0.305: R50.2 88.87,144.94 C20.1 88.87,143.61 86.45,141.19 79.46,141.19 78.19,139.28 78.19,117.69 109.31,86.58 110.58,86.58 111.21,85.94 111.21,80.23 110.58,79.59 v109.94,79.59 | 107.4,79.59 TEENSY3.2_1.27
S20-A19  (via drill 0.6)
  Top 0.305: v92.16,140.55 v99.78,140.55 | v109.31,92.29 109.31,90.39 108.04,89.12 106.77,89.12 105.98,88.33 105.98,83.36 TEENSY3.2_1.28
  Bottom 0.305: R52.2 97.45,145.52 C22.2 100.25,141.02 v99.78,140.55 | v92.16,140.55 80.1,140.55 78.83,138.65 78.83,118.33 104.86,92.29 v109.31,92.29
SCK_13  (via drill 0.6)
  Top 0.305: v42,69.43 50.25,77.69 60.41,77.69 v61.05,77.05
  Bottom 0.305: D13.3 20.53,85.18 36.28,69.43 v42,69.43 | v61.05,77.05 62.95,77.05 63.59,77.69 71.84,77.69 72.48,77.05 78.19,77.05 81.37,80.23 81.37,92.29 82,92.93 82,97.37 85.81,101.18 90.89,101.18 98.51,93.56 98.51,85.75 TEENSY3.2_1.13
SCL_29  (via drill 0.6)
  Top 0.305: v45.17,66.89 45.17,70.07 51.52,76.42 57.24,76.42 58.51,75.15 v58.51,74.51 | v102.32,77.24 101.05,75.78 v97.88,75.78
  Bottom 0.305: D6.3 25.61,77.56 36.28,66.89 v45.17,66.89 | v58.51,74.51 62.95,74.51 64.86,76.42 70.57,76.42 71.21,75.78 77.56,75.78 79.46,73.88 95.97,73.88 v97.88,75.78 | TEENSY3.2_1.29 104.67,82.13 104.23,82.13 102.32,80.23 v102.32,77.24
SDA_30  (via drill 0.6)
  Top 0.305: v43.9,68.16 43.9,70.07 50.89,77.05 58.51,77.05 v59.78,75.78 | v97.88,78.96 98.51,78.32 103.59,78.32 TEENSY3.2_1.30
  Bottom 0.305: D30.3 23.07,81.37 36.28,68.16 v43.9,68.16 | v59.78,75.78 62.95,75.78 64.22,77.05 71.21,77.05 71.84,76.42 78.83,76.42 82,79.59 82,91.66 82.64,92.29 82.64,96.74 86.45,100.55 90.26,100.55 97.88,92.93 v97.88,78.96
SOLENOIDE  (via drill 0.6)
  Top 0.305: JP4.1 80.17,109.37 78.83,110.71 78.83,120.87 81.37,123.41 v86.45,123.41
  Bottom 0.305: JP4.2 JP4.1 | QUANTUM_CONNECTOR.14 103.72,124.8 88.48,124.8 87.08,123.41 v86.45,123.41
TEENSY1-RX_TEENSY2-TX  (via drill 0.6)
  Top 0.305: QUANTUM_CONNECTOR.29 130.28,123.51 135.6,118.2 137.37,118.2 142.96,112.61 142.96,102.58 v144.23,101.31 | TEENSY3.2_1.0 115.66,54.83 142.96,54.83 144.23,56.1 v144.23,61.81 | v144.23,97.12 v144.23,75.78
  Bottom 0.305: v144.23,101.31 v144.23,97.12 | v144.23,75.78 v144.23,61.81
TEENSY1-TX_TEENSY2-RX  (via drill 0.6)
  Top 0.305: QUANTUM_CONNECTOR.30 129.9,126.05 135.34,120.61 137.37,120.61 145.76,112.23 v145.76,104.61 | v145.76,65.11 145.76,64.35 144.49,63.08 135.98,63.08 v135.47,63.46 | v145.76,95.34 v145.76,78.32 | v119.47,63.72 119.47,57.37 118.73,56.63 TEENSY3.2_1.1
  Bottom 0.305: 145.76,78.58 v145.76,78.32 v145.76,65.11 | v145.76,104.61 v145.76,95.34 | v135.47,63.46 135.09,63.08 120.1,63.08 v119.47,63.72
TX1-RX2  (via drill 0.6)
  Top 0.305: PX.TX 107.17,21.81 95.34,21.81 94.07,23.08 94.07,34.51 92.16,36.41 92.16,42.76 90.89,44.03 90.89,51.65 89.77,52.74 89.75,52.77 65.01,52.77 64.48,53.3 64.48,60.41 62.95,61.94 62.95,64.99 44.54,64.99 39.46,70.07 v39.46,71.97
  Bottom 0.305: SX.RX 26.72,108.17 30.57,108.17 33.11,105.63 33.11,75.15 36.28,71.97 v39.46,71.97
TX2-RX3  (via drill 0.6)
  Top 0.305: SX.TX 26.53,106.26 v37.55,106.26
  Bottom 0.305: v37.55,106.26 36.92,106.9 36.92,141.82 40.73,145.63 56.6,145.63 57.87,144.36 57.87,141.82 58.51,141.19 66.13,141.19 66.95,142.01 AX.RX
TX3-RX4  (via drill 0.6)
  Top 0.305: DX.RX v171.13,106.04 | v68.21,138.65 66.76,138.65 64.22,141.19 64.22,142.68 AX.TX | v71.21,138.65 81.37,138.65 82,138.01 106.77,138.01 107.4,138.65 135.98,138.65 140.42,134.2 140.42,132.93 v154.39,118.96
  Bottom 0.305: v71.21,138.65 v68.21,138.65 | v171.13,106.04 167.32,106.04 v154.39,118.96
US-AX  (via drill 0.6)
  Top 0.305: IC2.4 67.4,65.45 v67.4,68.16 | v62.32,148.81 66.76,148.81 69.3,146.27 69.3,143.05 AX.AN
  Bottom 0.305: v67.4,68.16 66.76,67.53 51.52,67.53 43.27,75.78 38.82,75.78 36.28,78.32 36.28,142.46 42.63,148.81 v62.32,148.81
US-DX  (via drill 0.6)
  Top 0.305: IC2.3 66.31,61.63 67.4,60.54 68.67,60.54 69.56,59.65 69.56,57.87 69.68,57.75 90.51,57.75 92.16,56.1 92.16,45.94 94.07,44.03 v94.07,42.76 | v182.33,66.26 178.52,62.45 165.82,62.45 165.19,62.45 150.58,47.84 102.32,47.84 101.69,47.21 v101.69,44.03 | v194.4,97.37 194.4,98.48 DX.AN
  Bottom 0.305: v182.33,66.26 182.33,80.86 174.71,88.48 174.71,92.29 177.25,94.83 191.86,94.83 v194.4,97.37 | v94.07,42.76 100.42,42.76 v101.69,44.03
US-PX  (via drill 0.6)
  Top 0.305: v95.34,28.16 95.34,34.51 92.8,37.05 92.8,43.4 91.53,44.67 91.53,54.95 91.21,55.27 67.33,55.27 67.02,55.46 67.02,59.91 65.04,61.88 IC2.2
  Bottom 0.305: v95.34,28.16 95.97,27.52 98.51,27.52 99.15,26.89 99.15,25.62 102.96,25.62 103.78,24.8 PX.AN
US-SIGNAL  (via drill 0.6)
  Top 0.305: 106.32,28.06 R4.2 106.64,23.49 PX.RX | TEENSY3.2_1.33 104.96,71.87 106.13,70.7 108.04,70.7 108.93,69.81 v108.93,68.16
  Bottom 0.305: v108.93,68.16 108.93,65.88 106.77,63.72 106.77,44.67 110.58,40.86 110.58,36.41 108.67,34.51 97.24,34.51 96.61,33.87 96.61,32.6 97.24,31.97 106.32,31.97 106.64,31.65 106.64,23.81 arc-90 PX.RX
US-SX  (via drill 0.6)
  Top 0.305: SX.AN 29.89,107.53 v39.46,107.53 | v64.86,73.24 65.04,73.43 IC2.23
  Bottom 0.305: v39.46,107.53 39.46,106.26 36.92,103.72 36.92,78.96 39.46,76.42 43.9,76.42 52.16,68.16 64.86,68.16 v64.86,73.24
VBAT  (via drill 0.6)
  Top 0.305: v191.86,68.16 v175.35,68.16 | v164.55,68.8 158.84,68.8 v158.2,68.16 | v151.22,68.16 146.77,72.61 140.64,72.61 R5.2
  Bottom 0.305: BATTERIA.1 193.03,69.34 v191.86,68.16 | v175.35,68.16 174.71,68.8 v164.55,68.8 | v158.2,68.16 v151.22,68.16
  Bottom 2.54: MAIN-SWITCH.2 193.71,75.34 BATTERIA.1
VIN  (via drill 0.6)
  Top 0.305: 99.78,51.46 TEENSY3.2_1.VIN 99.69,50.48 100.42,49.75 147.41,49.75 v148.04,50.38 | D1.A 170.27,73.81 170.27,70.7 153.12,53.56 v151.22,53.56
  Top 2.54: MAIN-SWITCH.1 202.07,80.8 200.75,82.13 184.24,82.13 | 184.24,82.13 183.48,82.13 D2.A | 184.24,82.13 184.24,80.23 179.1,75.09 SWITCH-MOT.2 171.55,75.09 D1.A
  Bottom 0.305: v148.04,50.38 v151.22,53.56
VMOT
  Top 2.54: SWITCH-MOT.1 178.32,80.23 174.08,80.23 170.93,83.37 PDX.VMOT-1 170.72,86.58 165.19,86.58 162.65,88.48 162.65,106.26 168.48,111.2 | ADX.VMOT-1 170.92,113.27 168.48,111.2 | ASX.VMOT-1 48.43,128.4 56.6,120.23 | 56.6,120.23 56.6,101.18 52.16,96.74 | 52.16,96.74 41.4,96.74 PSX.VMOT-1 52.07,96.65 52.16,96.74 | 56.6,120.23 56.6,147.54 61.05,151.98 77.56,151.98 83.91,145.63 134.05,145.63 168.48,111.2
VUSB  (via drill 0.6)
  Top 0.305: USB_2.1 79.46,35.4 v82.89,38.82
  Bottom 0.305: TEENSY3.2_1.VUSB 102.32,54.19 104.23,54.19 104.86,53.56 104.86,41.49 104.23,40.86 102.96,40.86 101.05,38.95 94.07,38.95 92.8,37.68 83.27,37.68 82.89,38.06 v82.89,38.82

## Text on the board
tPlace: 1 | 3 | 5 | 7 | 9 | 11 | 13 | 15 | 17 | 19 | 21 | 23 | 25 | 27 | 29 | 3.3 | 3.3 | 3.3 | 3.3 | GND | GND | GND | GND | Developed by: / Andrea Valeri / Emanuele Giacomini / Alessio Di Brigida / Fabio Ricci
